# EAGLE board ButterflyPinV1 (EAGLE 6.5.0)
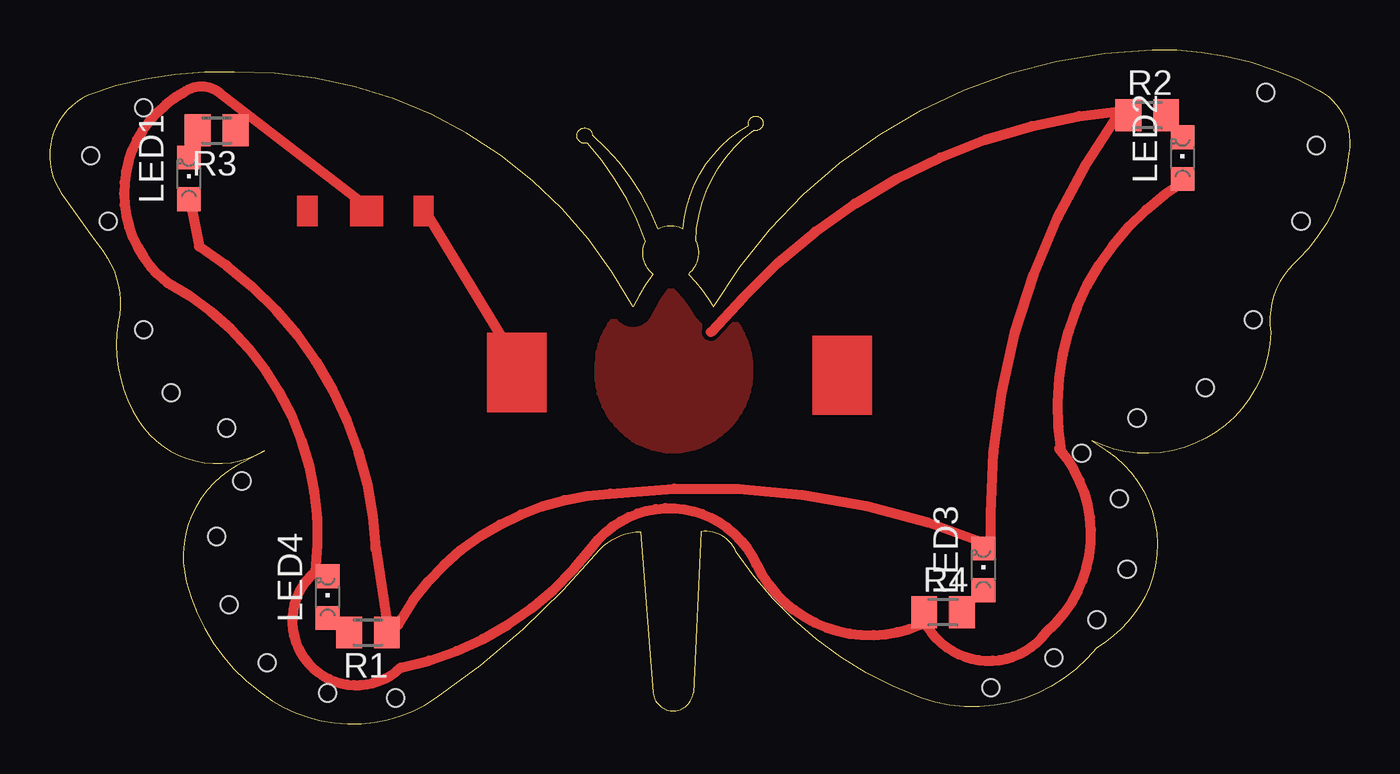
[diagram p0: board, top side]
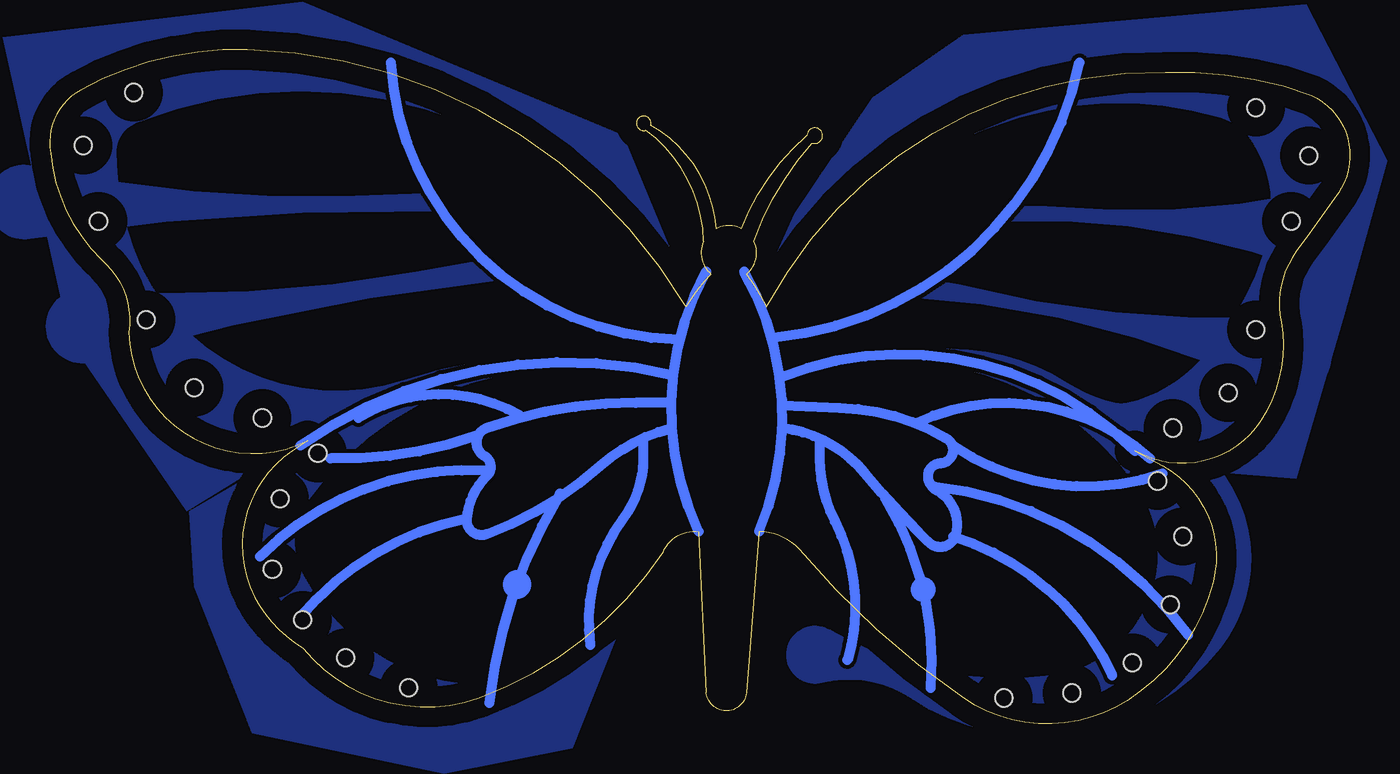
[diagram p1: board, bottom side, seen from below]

Size 65.48 x 33.94 mm. Coordinates in mm from the lower left corner, seen from the top.
Outline: 30.38,22.64 arc10 29.37,20.99 arc63 9.3,32.8 arc22 1.93,31.66 arc105 0.79,26.45 arc2 2.7,23.78 arc-48 3.46,20.23 arc42 4.47,15.27 arc88 10.82,13.75 9.43,12.99 arc76 6.89,7.15 arc43 11.21,1.18 arc67 19.46,1.3 arc16 27.72,8.8 arc-44 29.75,9.69 30.38,1.56 arc166 32.41,1.56 32.8,9.69 arc-72 34.57,8.67 arc36 43.84,1.3 arc70 52.73,3.84 arc32 55.15,6.38 arc84 53.24,13.75 52.48,14.26 arc115 61.5,19.72 arc-59 62.89,23.4 arc40 65.43,28.74 arc71 63.91,31.91 arc30 55.53,33.94 arc58 33.43,20.99 arc17 32.16,22.64 arc75 32.54,24.29 arc-53 35.46,29.88 arc301 35.21,30.13 arc56 31.91,24.93 arc56 30.64,24.93 arc28 27.33,29.62 arc288 27.08,29.24 arc-23 30,24.29 arc75 30.38,22.64
Copper layers (1*16): Top 0.035mm / dielectric 1.5mm / Bottom 0.035mm
Design rules "default": minimum track width 10mil, minimum drill 24mil, track to track 8mil, track to pad 8mil, pad to pad 8mil, via to via 8mil, smd to smd 8mil, copper to edge 40mil, drill to drill 8mil, minimum pad ring 10mil, minimum via ring 8mil, stop-mask expansion 4mil, vias tented up to drill 0mil, thermal gap 10mil
Holes 0.86 mm at 17.43,1.3 14,1.56 10.95,3.08 9.05,6 8.41,9.43 9.68,12.23 8.92,14.89 6.13,16.67 4.73,19.85 2.95,25.31 2.06,28.61 4.73,31.02 47.4,1.81 50.58,3.34 52.73,5.24 54.26,7.78 53.88,11.34 51.97,13.62 54.77,15.4 58.2,16.92 60.61,20.35 63.02,25.31 63.78,29.12 61.24,31.78

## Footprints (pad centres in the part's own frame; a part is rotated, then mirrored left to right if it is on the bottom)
CHIPLED_0805 = smd 1.2 x 1.2: A 0,-1.05; C 0,1.05
M0805 = smd 1.3 x 1.6: 1 -0.95,0; 2 0.95,0

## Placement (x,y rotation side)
LED1  [CHIPLED_0805]  7.01,27.47 0 top
LED2  [CHIPLED_0805]  57.05,28.48 0 top
LED3  [CHIPLED_0805]  47.02,7.78 0 top
LED4  [CHIPLED_0805]  14,6.38 0 top
R1  [M0805]  16.03,4.61 180 top
R2  [M0805]  55.27,30.64 0 top
R3  [M0805]  8.41,29.88 180 top
R4  [M0805]  44.99,5.62 0 top

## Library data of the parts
LED1-LED4 = led
R1-R4 = resistor

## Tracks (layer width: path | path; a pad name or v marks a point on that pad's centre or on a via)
S$1
  pour Top: 35.26,17.81 arc90 31.26,21.81 arc90 27.64,17.69 arc90 31.38,13.81 arc90
S$2
  Top 0.508: 23.78,17.81 19.08,25.56
S$3
  Top 0.508: 16.29,25.81 8.54,31.78 arc75 6.76,31.78 arc113 5.87,22.26 arc-69 13.36,7.65 arc183 17.68,2.83 arc42 27.33,8.92 arc-119 35.59,8.03 arc87 43.84,4.99 arc-80 44.23,4.86 arc110 50.19,4.61 arc90 50.83,13.88
S$4
  Top 0.508: 16.41,8.92 17.05,4.73
S$5
  Top 0.508: 17.56,4.99 18.32,6.26 arc-51 28.22,11.59 arc-29 47.27,9.05
S$6
  Top 0.508: 47.4,9.05 47.4,10.57 arc-36 53.88,30.77
S$7
  Top 0.508: 33.3,19.72 34.95,21.5 arc-42 54.26,30.89
S$8
  Top 0.508: 7.14,25.94 7.52,24.04 arc-56 16.41,8.8
S$10
  Bottom 0.508: 32.8,9.69 arc54 32.41,22.77
S$11
  Bottom 0.508: 52.86,14 arc49 34.07,17.56
S$12
  pour Bottom: 34.57,17.31 36.99,17.69 arc-63 52.48,11.21 arc-63 52.73,7.53 arc-101 36.99,4.22 39.15,-1.24 45.62,-2.51 55.27,-0.47 58.2,6.89 58.45,10.7 51.72,14.64 47.65,16.8 41.3,18.32 34.45,17.94 34.19,17.18
S$13
  Bottom 0.508: 33.81,19.34 arc85 48.29,33.31
S$14
  Bottom 0.508: 28.99,19.46 arc-73 13.62,33.31
S$15
  pour Bottom: 33.43,20.73 34.7,22.51 arc-76 61.12,30.26 arc-69 62.13,28.74 arc-19 61.24,23.91 arc-88 47.65,17.31 arc31 34.07,17.94 34.07,17.43 37.11,17.94 40.67,18.07 45.24,17.56 50.7,15.53 58.58,10.7 64.42,19.21 67.85,34.58 52.73,36.36 36.61,29.62 33.81,22.89 33.3,20.86
S$16
  Bottom 0.508: 34.19,16.16 35.97,16.16 arc-19 43.46,14.89 arc-131 43.59,13.5 arc106 43.46,12.48 arc-42 44.48,10.32 | 44.48,10.32 arc-115 43.46,9.56 arc-21 37.75,12.99 arc26 34.19,14.89 | 44.48,10.32 arc-39 52.86,5.37
S$17
  pour Bottom: 29.37,20.73 28.86,21.5 arc40 16.67,30.51 arc33 6.51,30.51 arc42 4.86,29.24 arc44 4.09,24.67 arc34 7.9,17.94 arc31 11.21,16.16 arc26 11.84,16.16 arc20 14.25,17.18 arc-28 19.21,18.83 arc-5 23.65,18.96 arc-20 28.6,17.69 26.57,18.45 25.05,18.58 21.49,18.7 17.81,18.07 14.89,16.8 9.17,12.86 2.7,12.35 0.28,20.61 -1.88,28.35 2.19,36.23 19.46,34.7 24.03,31.53 27.97,25.69 29.49,22.26
S$18
  Bottom 0.508: 28.6,16.04 25.68,15.91 arc29 20.35,14.38 arc150 20.6,13.11 arc-77 21.24,12.61 arc-76 20.73,11.72 arc72 19.84,9.56 arc128 21.24,9.18 21.75,9.69 arc5 24.41,12.61 arc-43 28.6,14.89
S$19
  Bottom 0.508: 35.59,14.26 35.59,13.37 arc37 36.61,10.32 arc-45 38.26,3.97
S$20
  Bottom 0.508: 26.7,14.13 26.7,13.37 arc-27 25.94,10.19 arc44 25.3,3.21
S$21
  Bottom 0.508: 29.75,9.69 arc-53 30.51,22.77
S$22
  Bottom 0.508: 10.82,13.75 arc-66 28.73,17.43
S$23
  pour Bottom: 28.48,17.31 26.45,17.81 arc68 10.82,12.1 arc118 15.02,2.45 arc38 26.19,4.73 arc-225 26.57,2.07 arc48 22.13,1.3 arc-86 6.51,3.84 arc-134 12.98,15.53 17.3,17.94 23.65,18.58 26.7,17.94
S$24
  Bottom 0.508: 39.78,11.59 arc-25 43.34,1.05
S$25
  Bottom 0.508: 23.4,11.34 arc36 21.11,1.81
S$26
  Bottom 0.508: 43.46,12.73 arc-49 54.89,8.42
S$27
  Bottom 0.508: 43.97,14.51 arc21 51.34,13.37
S$28
  Bottom 0.508: 41.81,15.53 arc-62 49.94,15.4
S$29
  Bottom 0.508: 19.97,9.43 arc48 11.97,2.45
S$30
  Bottom 0.508: 20.98,11.97 arc48 8.16,4.48
S$31
  Bottom 0.508: 19.97,14 arc-53 9.43,12.61
S$32
  Bottom 0.508: 21.87,15.15 arc67 10.06,13.37
S$33
  pour Bottom: 17.05,26.07 15.27,26.07 arc-17 2.32,26.7 arc216 1.93,22.77 arc-23 17.43,25.31 arc240 17.3,25.56 arc-166 17.05,25.69 arc107 16.79,26.07 arc6 16.67,26.07
  pour Bottom: 21.24,22.39 19.71,22.13 arc-17 3.84,20.48 arc216 3.46,16.54 arc-23 22.51,21.5 arc10 22.13,21.88 arc-166 21.37,22.13 arc107 20.98,22.39 arc6 20.98,22.13
S$34
  pour Bottom: 46.51,26.7 50.07,26.58 arc15 66.32,28.1 arc-202 66.45,24.42 arc10 45.88,25.81 46.38,26.7 46.64,26.7
  pour Bottom: 43.46,23.4 47.02,22.77 arc15 63.91,21.88 arc-202 63.02,18.32 arc10 42.45,22.39 43.72,23.53
S$35
  Top 0.508: 50.96,13.75 arc-68 57.18,27.34
(copper drawn outside any net)
  shapes: Bottom circle x2, Top area x5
